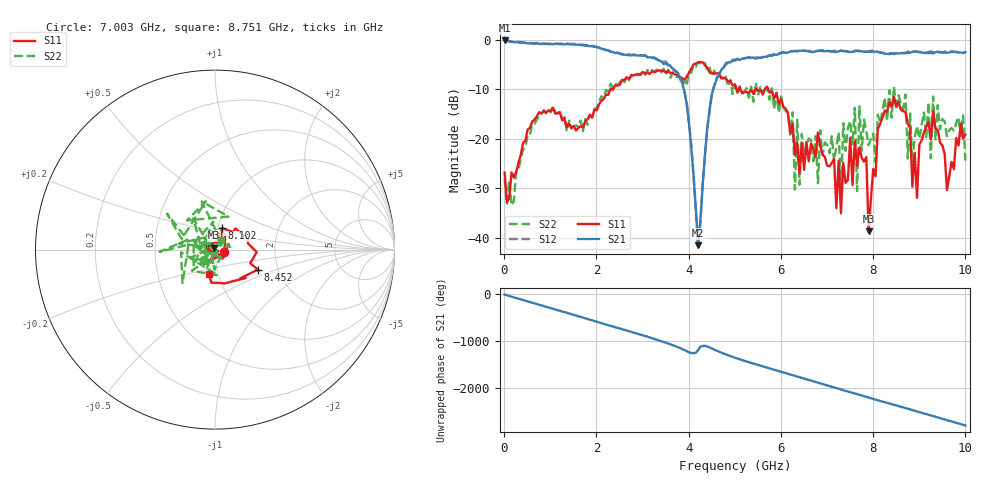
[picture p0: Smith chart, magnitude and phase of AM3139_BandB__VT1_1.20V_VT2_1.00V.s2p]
! Date/Time: Tue, Nov 13, 2018 4:59 PM
! Network Analyzer: Agilent Technologies E8364B Rev: A.07.50.67
! Sweep from 0.010 to 10.000 GHz, 201 Points, Sweep Type: LIN
! Power Supply: 1.200 V, 0.000 A
# Hz S DB R 50
!freq MagS11 AngS11 MagS21 AngS21 MagS12 AngS12 MagS22 AngS22
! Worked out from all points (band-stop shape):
!   201 points, 10 MHz to 10 GHz, reference 50 ohm
!   highest |S21| = -0.17 dB at 10 MHz (marker M1); lowest = -41.6 dB at 4.206 GHz (marker M2)
!   |S21| within 3 dB of the highest: start of sweep to 2.737 GHz; 5.826 GHz to end of sweep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
!   lowest |S11| = -38.8 dB at 7.902 GHz (marker M3), VSWR 1.02, Z = 49.4 + j0.991 ohm
!   |S11| at or under -10 dB: start of sweep to 2.303 GHz; 5.124 GHz to 5.45 GHz (325.7 MHz wide, 6.16 % of centre); 5.725 GHz to end of sweep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
!   |S22| runs from -33.5 to -4.6 dB; largest |S21 - S12| = 0.033
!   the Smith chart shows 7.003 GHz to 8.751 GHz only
!   S11 on the Smith chart (normalised r, x): 7.003 GHz: 1.11, -0.03; 8.102 GHz: 1.04, +0.25; 8.452 GHz: 1.58, -0.38; 8.751 GHz: 0.90, -0.25
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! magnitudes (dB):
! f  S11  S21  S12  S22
! 10 MHz  -26.9  -0.2  -0.2  -28.1
! 1.708 GHz  -17.8  -1.1  -1.1  -18.5
! 3.357 GHz  -6.2  -4.2  -4.2  -6.0
! 3.906 GHz  -8.1  -10.5  -10.4  -8.2
! 4.206 GHz  -4.7  -41.6  -41.7  -4.6
! 4.506 GHz  -6.8  -10.9  -10.8  -7.4
! 5.005 GHz  -9.1  -4.3  -4.0  -9.0
! 6.703 GHz  -22.1  -2.5  -2.3  -24.6
! 7.003 GHz  -25.4  -2.3  -2.3  -21.2
! 7.602 GHz  -20.5  -2.3  -2.2  -13.8
! 7.652 GHz  -25.5  -2.3  -2.2  -30.6
! 7.852 GHz  -23.7  -2.5  -2.4  -18.4
! 7.902 GHz  -38.8  -2.5  -2.4  -21.3
! 8.102 GHz  -18.1  -2.5  -2.5  -15.2
! 8.352 GHz  -12.7  -2.9  -2.8  -10.2
! 8.452 GHz  -11.6  -2.9  -2.8  -9.5
! 8.751 GHz  -17.0  -2.7  -2.4  -24.1
! 8.951 GHz  -32.0  -2.4  -2.5  -17.5
! 9.251 GHz  -20.2  -2.7  -2.4  -24.0
! 9.301 GHz  -14.4  -2.8  -2.6  -11.5
! 9.6 GHz  -30.4  -2.7  -2.4  -19.5
! 10 GHz  -19.2  -2.5  -2.4  -24.5
